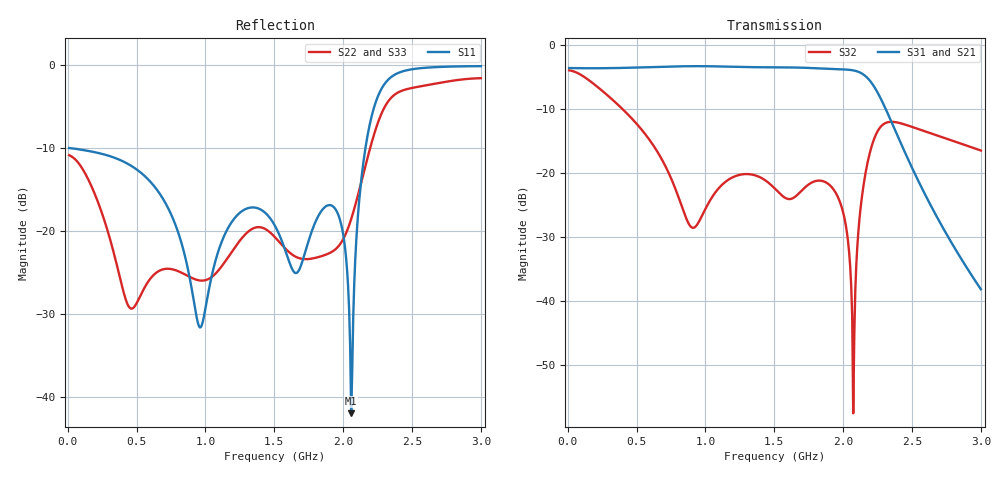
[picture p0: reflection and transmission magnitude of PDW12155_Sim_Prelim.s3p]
! Touchstone file exported from HFSS 2023.2.0
!  File:  P:/HFSS/Pierre/Quasi_PDW/PDW12155_12mil_vias.aedt
!  Generated:  3:53:05 PM  Sep 17, 2025
!  Design:  Design1
!  Project:  PDW12155_12mil_vias
!  Setup:  Setup1
!  Solution:  Sweep
! Variables:
!  Au_Thickness = 0.3mil
!  C1 = 0mil
!  C2 = -1mil
!  C3 = -1mil
!  L = 3mil
!  L1 = -1mil
!  L2 = 2mil
!  Poly_T = 0.2mil
!  RES = 50
!  T = 20mil
!  TopAu_Thickness = 0.3mil
!  Tune1 = 0mil
!  Tune2 = 1.5mil
!  Tune3 = 2mil
# GHz S MA R 50.000000
! Terminal data exported
! Port[1] = 1
! Port[2] = 2
! Port[3] = 3
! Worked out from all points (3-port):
!   401 points, 10 MHz to 3 GHz, reference 50 ohm
!   strongest paths, dB at 10 MHz, 757.5 MHz, 1.505 GHz, 2.252 GHz, 3 GHz:
!     S31: -3.7, -3.4, -3.5, -7.6, -38.2
!     S21: -3.7, -3.4, -3.5, -7.6, -38.2
!     S32: -4.0, -21.2, -22.5, -13.4, -16.5
!   lowest |S11| = -42.0 dB at 2.058 GHz (marker M1), VSWR 1.02, Z = 50.2 - j0.761 ohm
!   |S11| at or under -10 dB: start of sweep to 2.162 GHz
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0.01  0.3153 179.0  0.6555 -1.6  0.6563 -1.6
      0.6555 -1.6  0.2856 175.5  0.6304 -3.2
      0.6563 -1.6  0.6304 -3.2  0.2838 175.4
0.675275  0.164 121.7  0.6712 -104.9  0.6712 -104.9
          0.6712 -104.9  0.05806 -123.9  0.1315 -147.1
          0.6712 -104.9  0.1315 -147.1  0.05714 -122.9
0.959325  0.02621 161.2  0.6788 -153.0  0.6789 -153.0
          0.6788 -153.0  0.05026 -131.8  0.04265 59.3
          0.6789 -153.0  0.04265 59.3  0.04911 -130.6
1.505  0.1072 140.5  0.6647 106.0  0.6648 106.0
       0.6647 106.0  0.09159 -132.6  0.07489 -62.6
       0.6648 106.0  0.07489 -62.6  0.09043 -131.9
1.93855  0.1371 -91.0  0.6443 4.5  0.6443 4.5
         0.6443 4.5  0.07685 -71.0  0.07167 -83.4
         0.6443 4.5  0.07167 -83.4  0.07712 -69.9
2.05815  0.007974 -71.7  0.6335 -32.7  0.6333 -32.7
         0.6335 -32.7  0.1178 -39.2  0.01324 -112.7
         0.6333 -32.7  0.01324 -112.7  0.1187 -38.6
2.1329  0.2084 16.9  0.5976 -61.5  0.5974 -61.5
        0.5976 -61.5  0.1983 -29.1  0.06071 44.4
        0.5974 -61.5  0.06071 44.4  0.1995 -28.7
2.259975  0.6687 -36.1  0.4034 -115.2  0.4033 -115.2
          0.4034 -115.2  0.4663 -43.7  0.2192 -13.9
          0.4033 -115.2  0.2192 -13.9  0.4674 -43.5
2.47675  0.9327 -94.9  0.1236 -174.0  0.1236 -174.0
         0.1236 -174.0  0.7184 -91.3  0.2323 -79.1
         0.1236 -174.0  0.2323 -79.1  0.7184 -91.1
3  0.9811 -149.4  0.01226 131.1  0.01225 131.1
   0.01226 131.1  0.8305 -141.7  0.1488 -136.9
   0.01225 131.1  0.1488 -136.9  0.83 -141.5
